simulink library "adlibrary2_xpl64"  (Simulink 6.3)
undefined symbols (not defined in the file or in its folder): Bit, clock_ratio, Location, Lower, program, Width
libraries: xbsIndex_r4 x50, adlibrary2_xpl64 x1

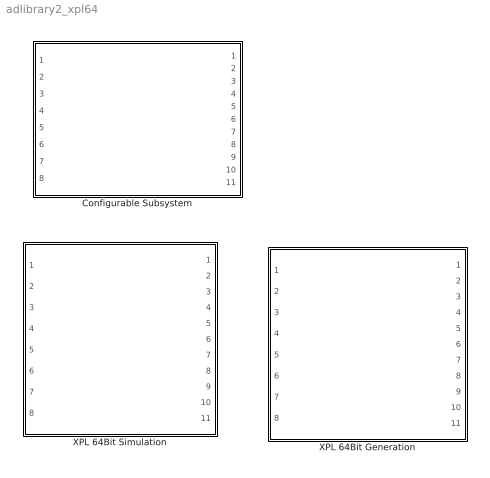
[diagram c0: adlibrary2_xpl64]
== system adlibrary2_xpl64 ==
  Configurable Subsystem : Subsystem  Tag=configX  BlockChoice=XPL 64Bit Simulation  mask{program=program, clock_ratio=clock_ratio}
      mask prompts: program "Local Bus Script Program"; clock_ratio "Clock Ratio"
  XPL 64Bit Generation : Subsystem
  XPL 64Bit Simulation : Subsystem  mask{program=program, clock_ratio=clock_ratio}
      mask prompts: program "Local Bus Script Program"; clock_ratio "Clock Ratio"

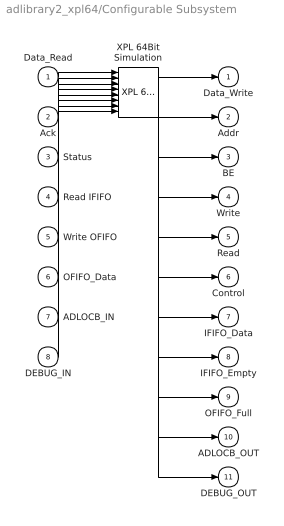
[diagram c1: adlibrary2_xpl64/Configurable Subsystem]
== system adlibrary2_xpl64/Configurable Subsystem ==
  Data_Read : Inport
  Ack : Inport  Port=2
  Status : Inport  Port=3
  Read IFIFO : Inport  Port=4
  Write OFIFO : Inport  Port=5
  OFIFO_Data : Inport  Port=6
  ADLOCB_IN : Inport  Port=7
  DEBUG_IN : Inport  Port=8
  XPL 64Bit Simulation : adlibrary2_xpl64/XPL 64Bit Simulation  program=program  clock_ratio=clock_ratio
  Data_Write : Outport
  Addr : Outport  Port=2
  BE : Outport  Port=3
  Write : Outport  Port=4
  Read : Outport  Port=5
  Control : Outport  Port=6
  IFIFO_Data : Outport  Port=7
  IFIFO_Empty : Outport  Port=8
  OFIFO_Full : Outport  Port=9
  ADLOCB_OUT : Outport  Port=10
  DEBUG_OUT : Outport  Port=11
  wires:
  Data_Read/1 -> XPL 64Bit Simulation/1
  Ack/1 -> XPL 64Bit Simulation/2
  Status/1 -> XPL 64Bit Simulation/3
  Read IFIFO/1 -> XPL 64Bit Simulation/4
  Write OFIFO/1 -> XPL 64Bit Simulation/5
  OFIFO_Data/1 -> XPL 64Bit Simulation/6
  ADLOCB_IN/1 -> XPL 64Bit Simulation/7
  DEBUG_IN/1 -> XPL 64Bit Simulation/8
  XPL 64Bit Simulation/1 -> Data_Write/1
  XPL 64Bit Simulation/2 -> Addr/1
  XPL 64Bit Simulation/3 -> BE/1
  XPL 64Bit Simulation/4 -> Write/1
  XPL 64Bit Simulation/5 -> Read/1
  XPL 64Bit Simulation/6 -> Control/1
  XPL 64Bit Simulation/7 -> IFIFO_Data/1
  XPL 64Bit Simulation/8 -> IFIFO_Empty/1
  XPL 64Bit Simulation/9 -> OFIFO_Full/1
  XPL 64Bit Simulation/10 -> ADLOCB_OUT/1
  XPL 64Bit Simulation/11 -> DEBUG_OUT/1

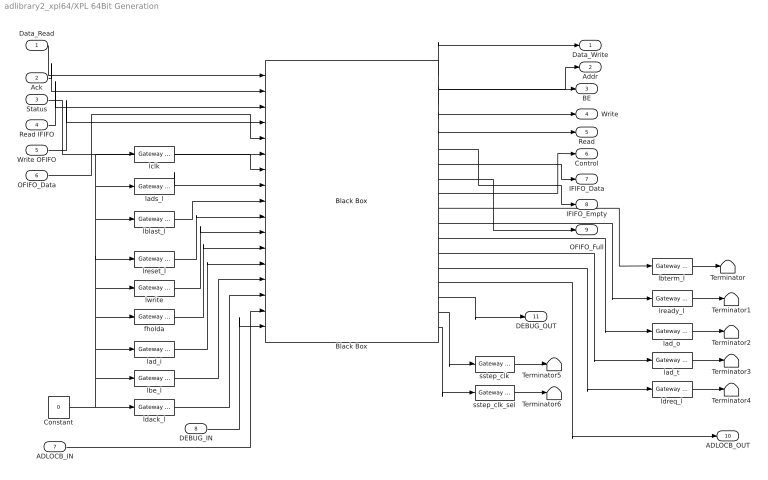
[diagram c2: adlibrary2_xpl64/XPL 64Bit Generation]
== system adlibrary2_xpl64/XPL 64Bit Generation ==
  Data_Read : Inport
  Ack : Inport  Port=2
  Status : Inport  Port=3
  Read IFIFO : Inport  Port=4
  Write OFIFO : Inport  Port=5
  OFIFO_Data : Inport  Port=6
  ADLOCB_IN : Inport  Port=7
  DEBUG_IN : Inport  Port=8
  Black Box : xbsIndex_r4/Black Box  init_code=lbif64_xpl_config  sim_method=Inactive  block_type=blackbox2
  Constant : Constant  Value=0
  Terminator{,1..6} (7 alike) : Terminator
  fholda : xbsIndex_r4/Gateway In  arith_type=Boolean  n_bits=8  bin_pt=6  period=1  dbl_ovrd=off  timing_constraint=None  locs_specified=off  LOCs={}  block_type=gatewayin
  lad_i : xbsIndex_r4/Gateway In  arith_type=Unsigned  n_bits=64  bin_pt=0  period=1  dbl_ovrd=off  timing_constraint=None  locs_specified=off  LOCs={}  block_type=gatewayin
  lad_o : xbsIndex_r4/Gateway Out  hdl_port=on  timing_constraint=None  locs_specified=off  LOCs={}  block_type=gatewayout
  lad_t : xbsIndex_r4/Gateway Out  hdl_port=on  timing_constraint=None  locs_specified=off  LOCs={}  block_type=gatewayout
  lads_l : xbsIndex_r4/Gateway In  arith_type=Boolean  n_bits=8  bin_pt=6  period=1  dbl_ovrd=off  timing_constraint=None  locs_specified=off  LOCs={}  block_type=gatewayin
  lbe_l : xbsIndex_r4/Gateway In  arith_type=Unsigned  n_bits=8  bin_pt=0  period=1  dbl_ovrd=off  timing_constraint=None  locs_specified=off  LOCs={}  block_type=gatewayin
  lblast_l : xbsIndex_r4/Gateway In  arith_type=Boolean  n_bits=8  bin_pt=6  period=1  dbl_ovrd=off  timing_constraint=None  locs_specified=off  LOCs={}  block_type=gatewayin
  lbterm_l : xbsIndex_r4/Gateway Out  hdl_port=on  timing_constraint=None  locs_specified=off  LOCs={}  block_type=gatewayout
  lclk : xbsIndex_r4/Gateway In  arith_type=Boolean  n_bits=8  bin_pt=6  period=1  dbl_ovrd=off  timing_constraint=None  locs_specified=off  LOCs={}  block_type=gatewayin
  ldack_l : xbsIndex_r4/Gateway In  arith_type=Unsigned  n_bits=2  bin_pt=0  period=1  dbl_ovrd=off  timing_constraint=None  locs_specified=off  LOCs={}  block_type=gatewayin
  ldreq_l : xbsIndex_r4/Gateway Out  hdl_port=on  timing_constraint=None  locs_specified=off  LOCs={}  block_type=gatewayout
  lready_l : xbsIndex_r4/Gateway Out  hdl_port=on  timing_constraint=None  locs_specified=off  LOCs={}  block_type=gatewayout
  lreset_l : xbsIndex_r4/Gateway In  arith_type=Boolean  n_bits=8  bin_pt=6  period=1  dbl_ovrd=off  timing_constraint=None  locs_specified=off  LOCs={}  block_type=gatewayin
  lwrite : xbsIndex_r4/Gateway In  arith_type=Boolean  n_bits=8  bin_pt=6  period=1  dbl_ovrd=off  timing_constraint=None  locs_specified=off  LOCs={}  block_type=gatewayin
  sstep_clk : xbsIndex_r4/Gateway Out  hdl_port=on  timing_constraint=None  locs_specified=off  LOCs={}  block_type=gatewayout
  sstep_clk_sel : xbsIndex_r4/Gateway Out  hdl_port=on  timing_constraint=None  locs_specified=off  LOCs={}  block_type=gatewayout
  Data_Write : Outport
  Addr : Outport  Port=2
  BE : Outport  Port=3
  Write : Outport  Port=4
  Read : Outport  Port=5
  Control : Outport  Port=6
  IFIFO_Data : Outport  Port=7
  IFIFO_Empty : Outport  Port=8
  OFIFO_Full : Outport  Port=9
  ADLOCB_OUT : Outport  Port=10
  DEBUG_OUT : Outport  Port=11
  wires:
  lbe_l/1 -> Black Box/14
  Data_Read/1 -> Black Box/1
  Ack/1 -> Black Box/2
  Status/1 -> Black Box/6
  Read IFIFO/1 -> Black Box/3
  Write OFIFO/1 -> Black Box/4
  OFIFO_Data/1 -> Black Box/5
  Black Box/1 -> Data_Write/1
  Black Box/2 -> Addr/1
  lclk/1 -> Black Box/7
  lads_l/1 -> Black Box/8
  lblast_l/1 -> Black Box/9
  lreset_l/1 -> Black Box/10
  lwrite/1 -> Black Box/11
  fholda/1 -> Black Box/12
  lad_i/1 -> Black Box/13
  ldack_l/1 -> Black Box/15
  Constant/1 -> ldack_l/1, lclk/1, lads_l/1, lblast_l/1, lreset_l/1, lwrite/1, fholda/1, lad_i/1, lbe_l/1
  lbterm_l/1 -> Terminator/1
  lready_l/1 -> Terminator1/1
  lad_o/1 -> Terminator2/1
  lad_t/1 -> Terminator3/1
  ldreq_l/1 -> Terminator4/1
  Black Box/14 -> ldreq_l/1
  Black Box/3 -> BE/1
  Black Box/4 -> Write/1
  Black Box/5 -> Read/1
  Black Box/6 -> IFIFO_Empty/1
  Black Box/7 -> IFIFO_Data/1
  Black Box/8 -> OFIFO_Full/1
  Black Box/9 -> Control/1
  Black Box/10 -> lbterm_l/1
  Black Box/11 -> lready_l/1
  Black Box/12 -> lad_o/1
  Black Box/13 -> lad_t/1
  Black Box/15 -> ADLOCB_OUT/1
  ADLOCB_IN/1 -> Black Box/16
  sstep_clk/1 -> Terminator5/1
  sstep_clk_sel/1 -> Terminator6/1
  DEBUG_IN/1 -> Black Box/17
  Black Box/17 -> sstep_clk/1
  Black Box/18 -> sstep_clk_sel/1
  Black Box/16 -> DEBUG_OUT/1

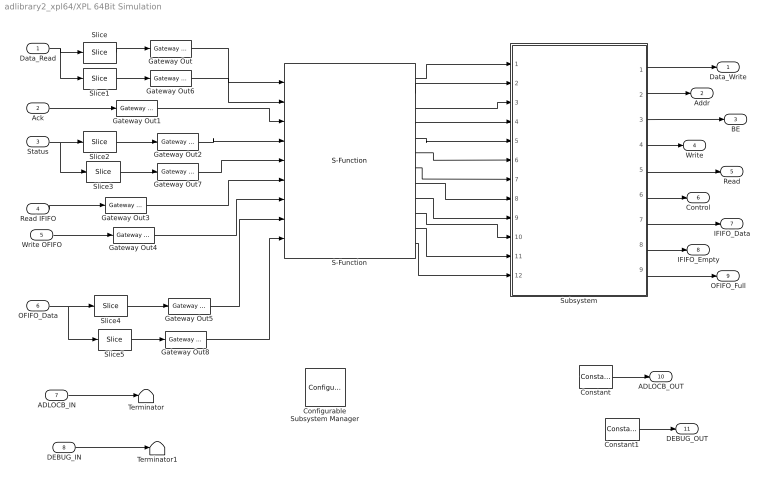
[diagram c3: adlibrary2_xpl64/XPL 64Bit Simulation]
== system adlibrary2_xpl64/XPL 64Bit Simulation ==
  Data_Read : Inport
  Ack : Inport  Port=2
  Status : Inport  Port=3
  Read IFIFO : Inport  Port=4
  Write OFIFO : Inport  Port=5
  OFIFO_Data : Inport  Port=6
  ADLOCB_IN : Inport  Port=7
  DEBUG_IN : Inport  Port=8
  Configurable Subsystem Manager : xbsIndex_r4/Configurable Subsystem Manager  Tag=xcfgMgr  block_type=configsubsys
  Constant : xbsIndex_r4/Constant  arith_type=Unsigned  const=0  n_bits=66  bin_pt=0  explicit_period=on  period=1  equ=P=C  opselect=C  inp2=PCIN>>17  opr=+  inp1=P  carry=CIN  dbl_ovrd=off  block_type=constant
  Constant1 : xbsIndex_r4/Constant  arith_type=Unsigned  const=0  n_bits=40  bin_pt=0  explicit_period=on  period=1  equ=P=C  opselect=C  inp2=PCIN>>17  opr=+  inp1=P  carry=CIN  dbl_ovrd=off  block_type=constant
  Gateway Out{,1..8} (9 alike) : xbsIndex_r4/Gateway Out  hdl_port=off  timing_constraint=None  locs_specified=off  LOCs={}  block_type=gatewayout
  S-Function : S-Function  FunctionName=lbif_xpl64  Parameters=program,clock_ratio
  Slice : xbsIndex_r4/Slice  nbits=32  boolean_output=off  mode=Lower Bit Location + Width  bit1=0  base1=MSB of Input  bit0=0  base0=LSB of Input  dbl_ovrd=off  block_type=slice
  Slice1 : xbsIndex_r4/Slice  nbits=32  boolean_output=off  mode=Lower Bit Location + Width  bit1=0  base1=MSB of Input  bit0=32  base0=LSB of Input  dbl_ovrd=off  block_type=slice
  Slice2 : xbsIndex_r4/Slice  nbits=32  boolean_output=off  mode=Lower Bit Location + Width  bit1=0  base1=MSB of Input  bit0=0  base0=LSB of Input  dbl_ovrd=off  block_type=slice
  Slice3 : xbsIndex_r4/Slice  nbits=32  boolean_output=off  mode=Lower Bit Location + Width  bit1=0  base1=MSB of Input  bit0=32  base0=LSB of Input  dbl_ovrd=off  block_type=slice
  Slice4 : xbsIndex_r4/Slice  nbits=32  boolean_output=off  mode=Lower Bit Location + Width  bit1=0  base1=MSB of Input  bit0=0  base0=LSB of Input  dbl_ovrd=off  block_type=slice
  Slice5 : xbsIndex_r4/Slice  nbits=32  boolean_output=off  mode=Lower Bit Location + Width  bit1=0  base1=MSB of Input  bit0=32  base0=LSB of Input  dbl_ovrd=off  block_type=slice
  Subsystem : Subsystem
  Terminator : Terminator
  Terminator1 : Terminator
  Data_Write : Outport
  Addr : Outport  Port=2
  BE : Outport  Port=3
  Write : Outport  Port=4
  Read : Outport  Port=5
  Control : Outport  Port=6
  IFIFO_Data : Outport  Port=7
  IFIFO_Empty : Outport  Port=8
  OFIFO_Full : Outport  Port=9
  ADLOCB_OUT : Outport  Port=10
  DEBUG_OUT : Outport  Port=11
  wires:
  Data_Read/1 -> Slice/1, Slice1/1
  Ack/1 -> Gateway Out1/1
  Status/1 -> Slice2/1, Slice3/1
  Read IFIFO/1 -> Gateway Out3/1
  Write OFIFO/1 -> Gateway Out4/1
  OFIFO_Data/1 -> Slice4/1, Slice5/1
  Slice/1 -> Gateway Out/1
  Slice1/1 -> Gateway Out6/1
  Gateway Out/1 -> S-Function/1
  Gateway Out6/1 -> S-Function/2
  Gateway Out1/1 -> S-Function/3
  Slice2/1 -> Gateway Out2/1
  Slice3/1 -> Gateway Out7/1
  Gateway Out2/1 -> S-Function/4
  Gateway Out7/1 -> S-Function/5
  Gateway Out3/1 -> S-Function/6
  Gateway Out4/1 -> S-Function/7
  Slice4/1 -> Gateway Out5/1
  Slice5/1 -> Gateway Out8/1
  Gateway Out5/1 -> S-Function/8
  Gateway Out8/1 -> S-Function/9
  S-Function/1 -> Subsystem/1(data_write0)
  S-Function/2 -> Subsystem/2(data_write1)
  S-Function/3 -> Subsystem/3(addr)
  S-Function/4 -> Subsystem/4(be)
  S-Function/5 -> Subsystem/5(write)
  S-Function/6 -> Subsystem/6(read)
  S-Function/7 -> Subsystem/7(control0)
  S-Function/8 -> Subsystem/8(control1)
  S-Function/9 -> Subsystem/9(ififo_data0)
  S-Function/12 -> Subsystem/12(ofifo_full)
  S-Function/11 -> Subsystem/11(ififo_empty)
  S-Function/10 -> Subsystem/10(ififo_data1)
  Subsystem/9(Out9) -> OFIFO_Full/1
  Subsystem/8(Out8) -> IFIFO_Empty/1
  Subsystem/7(Out7) -> IFIFO_Data/1
  Subsystem/6(Out6) -> Control/1
  Subsystem/5(Out5) -> Read/1
  Subsystem/4(Out4) -> Write/1
  Subsystem/3(Out3) -> BE/1
  Subsystem/2(Out2) -> Addr/1
  Subsystem/1(Out1) -> Data_Write/1
  ADLOCB_IN/1 -> Terminator/1
  Constant/1 -> ADLOCB_OUT/1
  DEBUG_IN/1 -> Terminator1/1
  Constant1/1 -> DEBUG_OUT/1

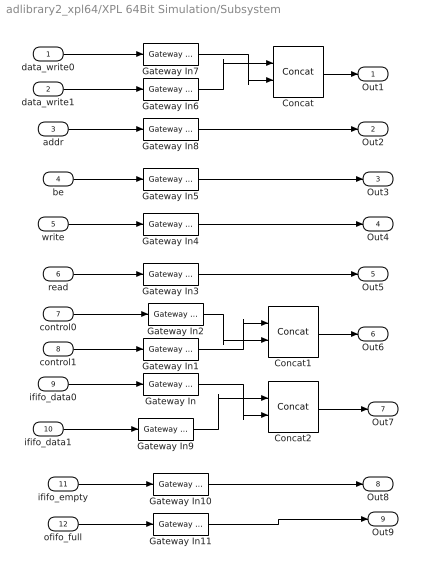
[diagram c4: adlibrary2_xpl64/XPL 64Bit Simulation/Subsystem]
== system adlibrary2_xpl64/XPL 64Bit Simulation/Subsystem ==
  data_write0 : Inport
  data_write1 : Inport  Port=2
  addr : Inport  Port=3
  be : Inport  Port=4
  write : Inport  Port=5
  read : Inport  Port=6
  control0 : Inport  Port=7
  control1 : Inport  Port=8
  ififo_data0 : Inport  Port=9
  ififo_data1 : Inport  Port=10
  ififo_empty : Inport  Port=11
  ofifo_full : Inport  Port=12
  Concat : xbsIndex_r4/Concat  num_inputs=2  dbl_ovrd=off  block_type=concat
  Concat1 : xbsIndex_r4/Concat  num_inputs=2  dbl_ovrd=off  block_type=concat
  Concat2 : xbsIndex_r4/Concat  num_inputs=2  dbl_ovrd=off  block_type=concat
  Gateway In{,1..2,6..7,9} (6 alike) : xbsIndex_r4/Gateway In  arith_type=Unsigned  n_bits=32  bin_pt=0  period=1  dbl_ovrd=off  timing_constraint=None  locs_specified=off  LOCs={}  block_type=gatewayin
  Gateway In10 : xbsIndex_r4/Gateway In  arith_type=Boolean  n_bits=8  bin_pt=6  period=1  dbl_ovrd=off  timing_constraint=None  locs_specified=off  LOCs={}  block_type=gatewayin
  Gateway In11 : xbsIndex_r4/Gateway In  arith_type=Boolean  n_bits=8  bin_pt=6  period=1  dbl_ovrd=off  timing_constraint=None  locs_specified=off  LOCs={}  block_type=gatewayin
  Gateway In3 : xbsIndex_r4/Gateway In  arith_type=Boolean  n_bits=32  bin_pt=0  period=1  dbl_ovrd=off  timing_constraint=None  locs_specified=off  LOCs={}  block_type=gatewayin
  Gateway In4 : xbsIndex_r4/Gateway In  arith_type=Boolean  n_bits=8  bin_pt=6  period=1  dbl_ovrd=off  timing_constraint=None  locs_specified=off  LOCs={}  block_type=gatewayin
  Gateway In5 : xbsIndex_r4/Gateway In  arith_type=Unsigned  n_bits=8  bin_pt=0  period=1  dbl_ovrd=off  timing_constraint=None  locs_specified=off  LOCs={}  block_type=gatewayin
  Gateway In8 : xbsIndex_r4/Gateway In  arith_type=Unsigned  n_bits=16  bin_pt=0  period=1  dbl_ovrd=off  timing_constraint=None  locs_specified=off  LOCs={}  block_type=gatewayin
  Out1 : Outport
  Out2 : Outport  Port=2
  Out3 : Outport  Port=3
  Out4 : Outport  Port=4
  Out5 : Outport  Port=5
  Out6 : Outport  Port=6
  Out7 : Outport  Port=7
  Out8 : Outport  Port=8
  Out9 : Outport  Port=9
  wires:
  data_write0/1 -> Gateway In7/1
  data_write1/1 -> Gateway In6/1
  be/1 -> Gateway In5/1
  write/1 -> Gateway In4/1
  read/1 -> Gateway In3/1
  control0/1 -> Gateway In2/1
  control1/1 -> Gateway In1/1
  ififo_data0/1 -> Gateway In/1
  addr/1 -> Gateway In8/1
  Gateway In6/1 -> Concat/1
  Gateway In7/1 -> Concat/2
  Concat/1 -> Out1/1
  Gateway In8/1 -> Out2/1
  Gateway In5/1 -> Out3/1
  Gateway In4/1 -> Out4/1
  Gateway In3/1 -> Out5/1
  Gateway In2/1 -> Concat1/2
  Gateway In1/1 -> Concat1/1
  Concat1/1 -> Out6/1
  ififo_data1/1 -> Gateway In9/1
  ififo_empty/1 -> Gateway In10/1
  ofifo_full/1 -> Gateway In11/1
  Gateway In9/1 -> Concat2/1
  Gateway In/1 -> Concat2/2
  Concat2/1 -> Out7/1
  Gateway In10/1 -> Out8/1
  Gateway In11/1 -> Out9/1
